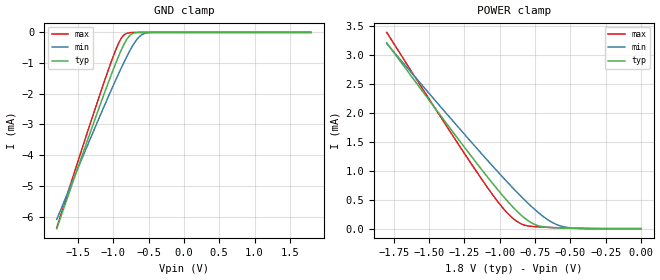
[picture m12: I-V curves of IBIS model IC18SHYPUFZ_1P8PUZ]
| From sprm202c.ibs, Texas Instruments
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|   Model IC18SHYPUFZ_1P8PUZ
[Model]   IC18SHYPUFZ_1P8PUZ
Model_type   Input
Polarity   Non-Inverting
Vinl =   0.8400V
Vinh =   0.9800V
C_comp   0.8000pF   0.9300pF   0.6600pF
[Model Spec]
|   typ   min   max
Vinh   0.98V   0.86V   1.05V
Vinl   0.84V   0.70V   0.91V
[Temperature Range]   25.0000   0.1250k   -40.0000
[Voltage Range]   1.8000V   1.6200V   1.9500V
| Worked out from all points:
|   GND clamp passes 1 mA (typ) near -0.96 V on its own axis
|   POWER clamp passes 1 mA (typ) near -1.12 V on its own axis
[GND_clamp]
| voltage   I(typ)   I(min)   I(max)
-1.8V     -6.396mA   -6.096mA   -6.371mA
-1.4V     -3.747mA   -3.876mA   -3.494mA
-1.08V    -1.698mA   -2.149mA   -1.29mA
-1V       -1.212mA   -1.731mA   -780.1uA
-920mV    -753.2uA   -1.325mA   -331.9uA
-880mV    -541.6uA   -1.127mA   -164uA
-840mV    -351uA     -935.1uA   -63.92uA
-760mV    -87.21uA   -575.2uA   -7.145uA
-680mV    -10.27uA   -272.4uA   -371.9nA
-600mV    -869.9nA   -79.49uA   -20.18nA
-520mV    -54.62nA   -13.17uA   -11.86nA
1.8V      239.3pA    20.15nA    226.6pA
[POWER_clamp]
| voltage   I(typ)   I(min)   I(max)
-1.8V     3.211mA    3.198mA    3.391mA
-1.4V     1.892mA    2.053mA    1.861mA
-1.14V    1.058mA    1.326mA    897.9uA
-1V       631.4uA    945.7uA    423uA
-940mV    460.8uA    787.6uA    254.6uA
-900mV    354.9uA    684.5uA    165uA
-840mV    215.1uA    534.5uA    73.55uA
-760mV    81.3uA     348.1uA    36.08uA
-660mV    22.21uA    154.2uA    23.26uA
-580mV    12.7uA     54.64uA    15.31uA
-440mV    4.715uA    5.192uA    5.044uA
0V        239.3pA    211.3pA    274pA
